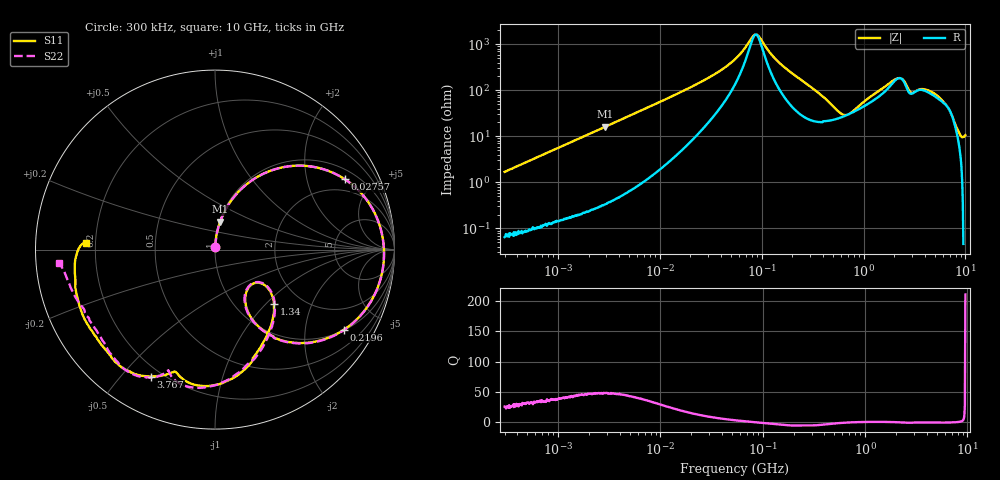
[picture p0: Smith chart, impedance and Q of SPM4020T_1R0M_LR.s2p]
! S-Parameter Data Generated by TDK Corporation
! Copyright(C) 2019 TDK Corporation.
! All Rights Reserved.
! TDK P/N: SPM4020T-1R0M-LR (Inductor)
! Property: L=1uH at 100kHz
! Size(LxWxT): 4.4x4.1x2mm
! Model Type: s2p (Touchstone File Format Version 1.0)
! Frequency: DC=Yes Start=0.3MHz Stop=10000MHz 802points Log-sweep
! Model Generated on Sep. 23, 2019
! Port Assignments:
!  1 ---@@@--- 2
! Applicable Conditions:
!  Temperature = 25 degC
!  DC Bias Current = 0 A
!  Small Signal Operation
! Terms and conditions regarding TDK Simulation Models
! (1)This simulation model is being provided solely for informational purposes. Please refer to the specifications of the products in terms of detailed characteristics of such products.
! (2)In no event shall TDK Corporation of any of its subsidiaries be liable for any loss or damage arising, directly or indirectly,
!  From any information contained in this simulation model, including, but not limited to loss or damages arising from any inaccuracies, omissions or errors in connection with such information.
! (3)Any and all copyrights on this simulation model are owned by TDK Corporation.
!  Duplication or redistribution of this simulation model without prior written permission from TDK Corporation is prohibited.
! (4)This simulation model is subject to any modification or change without any prior notice.
! (5)Neither TDK Corporation nor any of its subsidiaries shall make any warranty, express or implied,
!  Including but not limited to the correctness, implied warranties of merchantability and fitness for a particular purpose with respect to this simulation models.
! (6)The use of this simulation model shall be deemed to have consented to the terms and conditions hereof.
# Hz S MA R 50
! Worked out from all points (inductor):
!   801 points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, 300 kHz to 10 GHz, reference 50 ohm
!   read as one part in series: L = 895 nH near 318.3 kHz
!   highest Q = 48.5 at 2.928 MHz (marker M1), where L = 881 nH
!   self-resonance near 87.85 MHz
!   S11 on the Smith chart (normalised r, x): 300 kHz: 1.00, +0.03; 27.57 MHz: 1.41, +3.42; 219.6 MHz: 1.02, -3.21; 1.34 GHz: 1.47, -1.12; 3.767 GHz: 0.16, -0.60; 10 GHz: 0.16, +0.02
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300000  0.01668 87.0  0.9993 -1.0  0.9992 -1.0  0.01649 86.6
1713600  0.09403 83.3  0.9935 -5.5  0.9936 -5.4  0.09404 83.3
2927527  0.1587 79.6  0.984 -9.2  0.9841 -9.2  0.1586 79.6
9671944  0.4659 60.0  0.8694 -28.1  0.8695 -28.1  0.4658 60.0
2.756802e7  0.8237 28.4  0.4932 -56.1  0.4932 -56.1  0.8237 28.3
5.477226e7  0.9261 8.8  0.1966 -64.6  0.1966 -64.7  0.926 8.8
8.857507e7  0.9424 -3.5  0.0577 -0.2  0.05771 -0.2  0.9424 -3.6
1.454054e8  0.9186 -17.4  0.2172 56.6  0.2172 56.6  0.9185 -17.6
2.195581e8  0.846 -31.8  0.4078 48.2  0.4078 48.2  0.8458 -32.1
3.126428e8  0.7188 -46.4  0.5786 33.2  0.5786 33.2  0.7183 -46.7
4.687561e8  0.4928 -60.5  0.7198 10.3  0.7198 10.3  0.4914 -60.8
6.325141e8  0.3305 -59.3  0.752 -8.9  0.752 -8.9  0.3272 -59.8
8.414386e8  0.2842 -42.1  0.7132 -27.7  0.7132 -27.7  0.2807 -42.0
1.339606e9  0.4478 -42.8  0.5273 -58.8  0.5274 -58.8  0.4444 -41.7
1.767019e9  0.575 -61.3  0.3485 -73.6  0.3485 -73.7  0.5784 -60.2
2.446702e9  0.7575 -91.2  0.2202 -59.0  0.2202 -59.1  0.7636 -92.2
2.96667e9  0.7161 -107.6  0.2821 -62.9  0.2821 -62.9  0.7323 -110.3
3.766866e9  0.7921 -116.8  0.2129 -75.0  0.2129 -75.0  0.7824 -115.0
4.982529e9  0.8374 -128.5  0.1955 -76.7  0.1955 -76.8  0.8358 -126.0
6.333834e9  0.8251 -139.1  0.1952 -91.2  0.1953 -91.3  0.8045 -141.9
8.09931e9  0.806 -165.0  0.1678 -114.4  0.1679 -114.5  0.8314 -165.3
1e10  0.7211 177.2  0.127 -126.3  0.1271 -126.5  0.8738 -175.1
